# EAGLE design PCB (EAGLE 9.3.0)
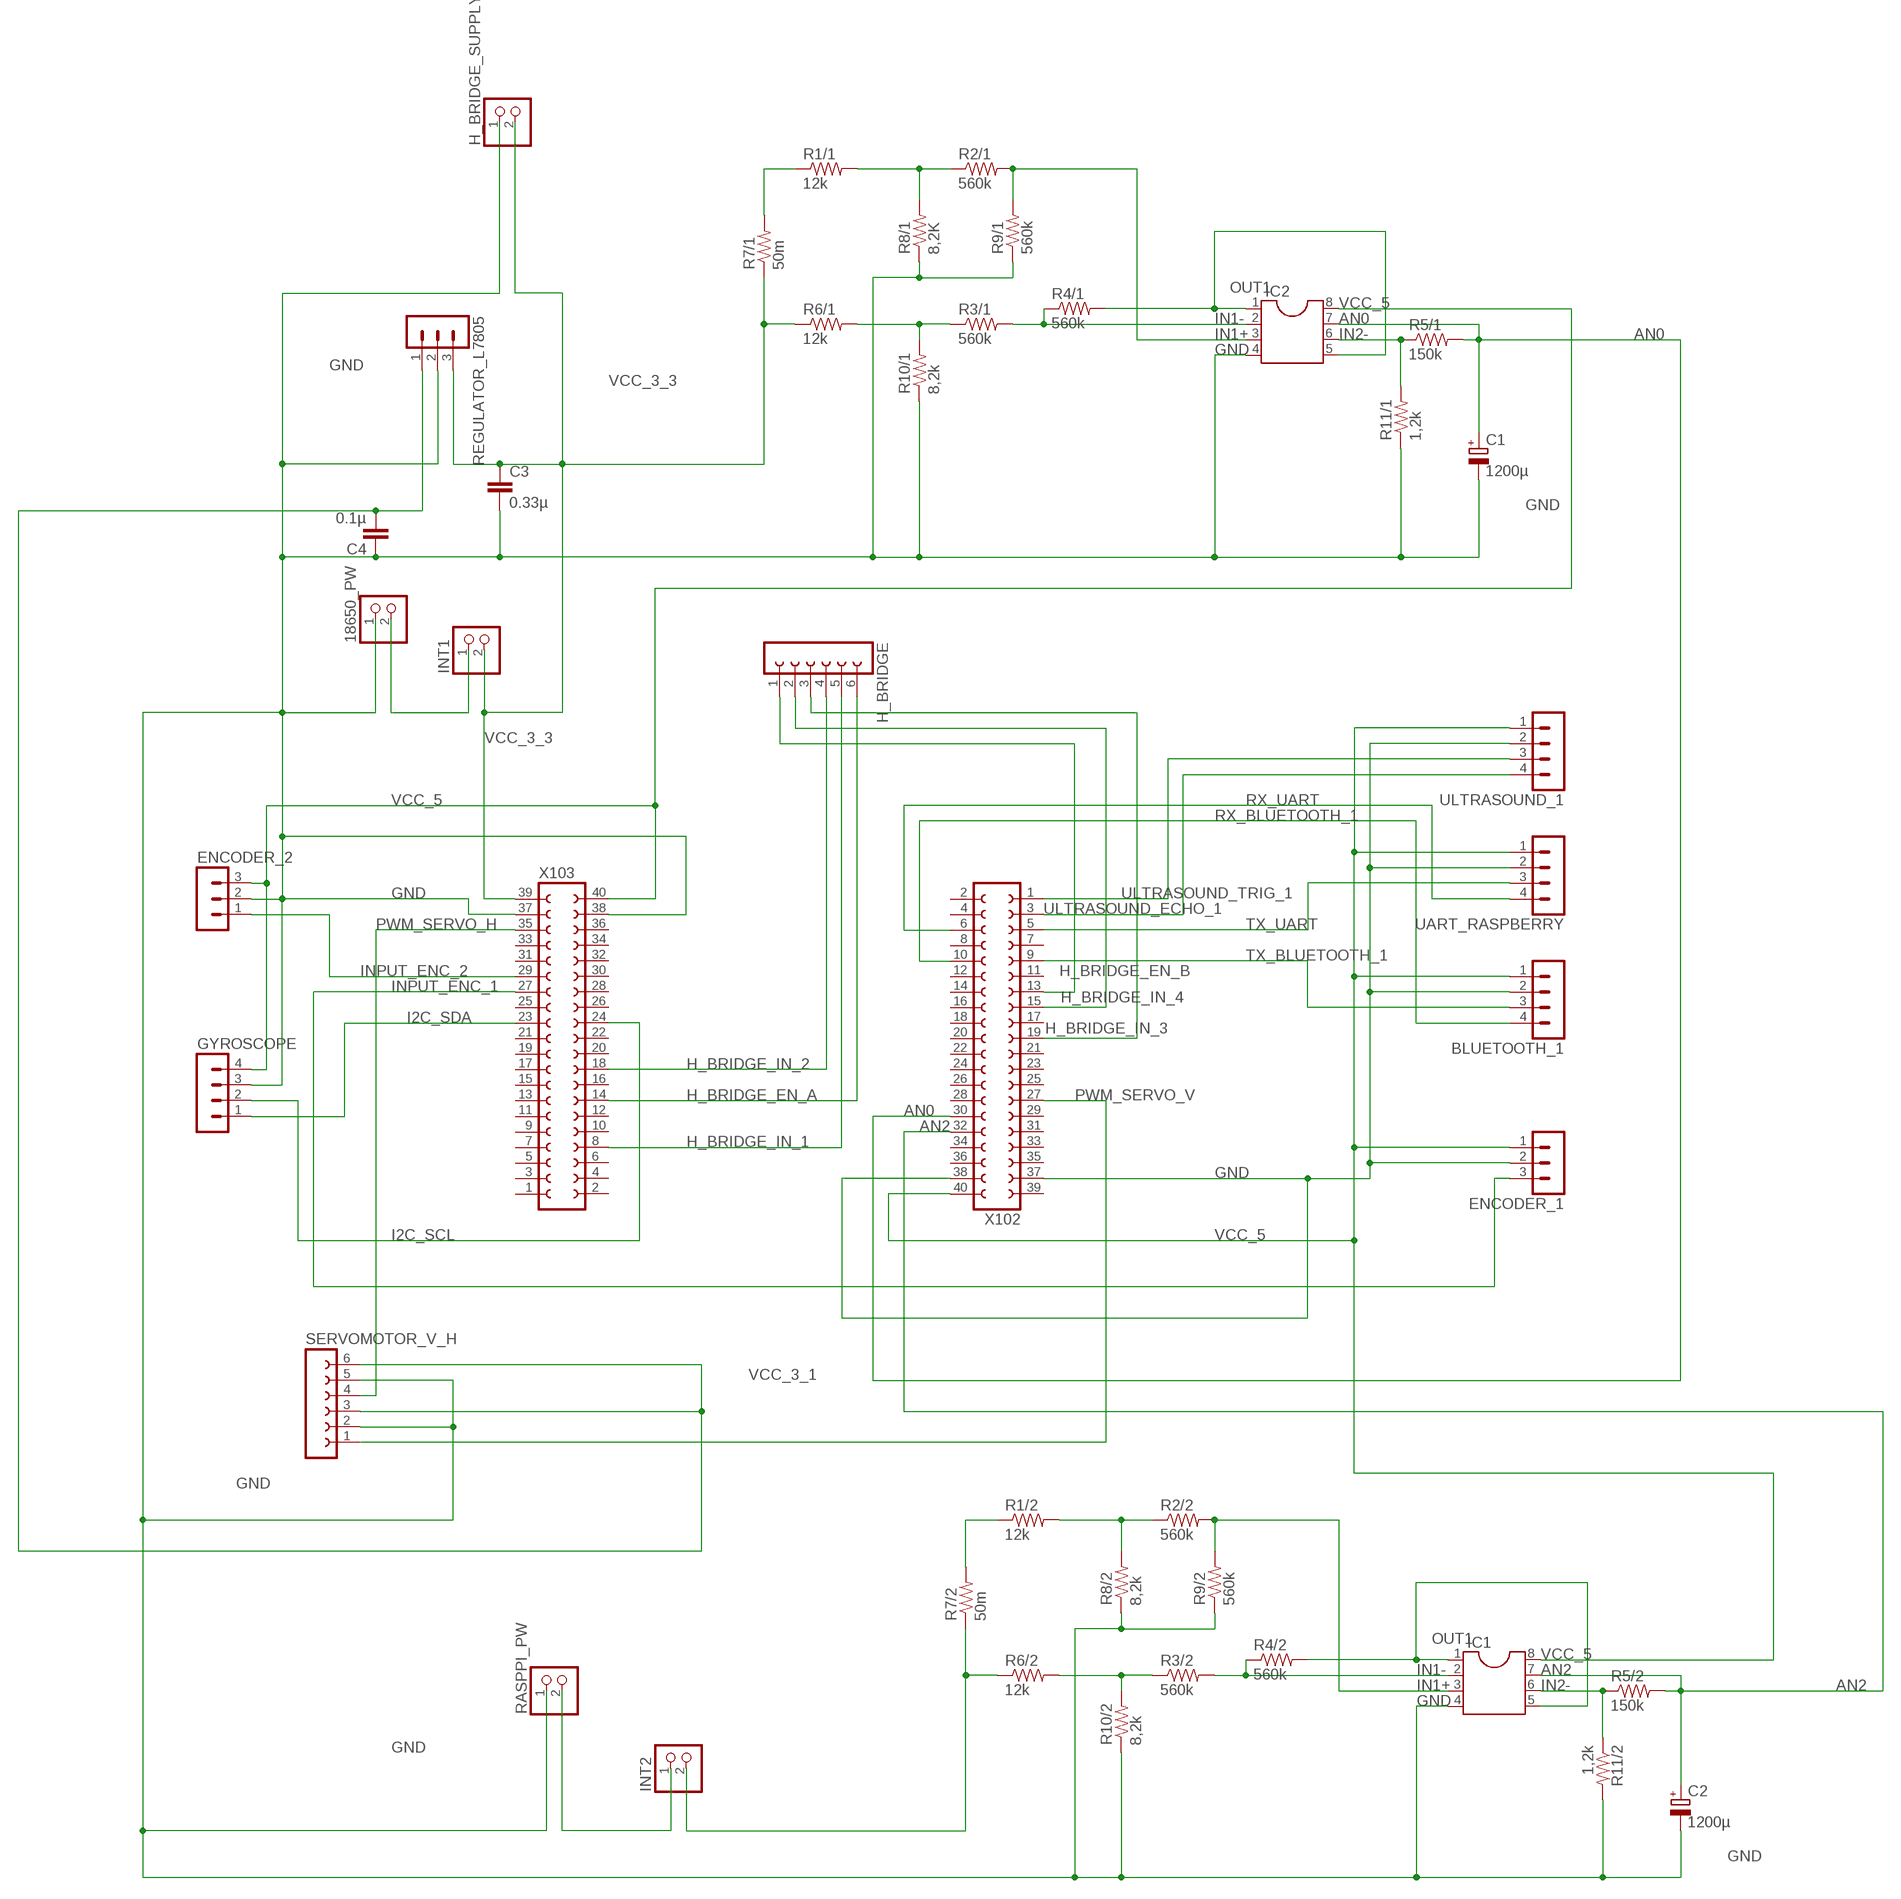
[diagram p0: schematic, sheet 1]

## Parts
18650_PW  PINHD-1X2  [1X02]
BLUETOOTH_1  MA04-1  [MA04-1]
C1  1200µ  CPOL-EUE2-5  [E2-5]
C2  1200µ  CPOL-EUE2-5  [E2-5]
C3  0.33µ  C-EU025-025X050  [C025-025X050]
C4  0.1µ  C-EU025-025X050  [C025-025X050]
ENCODER_1  MA03-1  [MA03-1]
ENCODER_2  MA03-1  [MA03-1]
GYROSCOPE  MA04-1  [MA04-1]
H_BRIDGE  FE06-1  [FE06]
H_BRIDGE_SUPPLY  PINHD-1X2  [1X02]
IC1  DIL8  [DIL08]
IC2  DIL8  [DIL08]
INT1  PINHD-1X2  [1X02]
INT2  PINHD-1X2  [1X02]
R1/1  12k  R-US_0207/10  [0207/10]
R1/2  12k  R-US_0207/10  [0207/10]
R2/1  560k  R-US_0207/10  [0207/10]
R2/2  560k  R-US_0207/10  [0207/10]
R3/1  560k  R-US_0207/10  [0207/10]
R3/2  560k  R-US_0207/10  [0207/10]
R4/1  560k  R-US_0207/10  [0207/10]
R4/2  560k  R-US_0207/10  [0207/10]
R5/1  150k  R-US_0207/10  [0207/10]
R5/2  150k  R-US_0207/10  [0207/10]
R6/1  12k  R-US_0207/10  [0207/10]
R6/2  12k  R-US_0207/10  [0207/10]
R7/1  50m  R-US_0207/10  [0207/10]
R7/2  50m  R-US_0207/10  [0207/10]
R8/1  8,2K  R-US_0207/10  [0207/10]
R8/2  8,2k  R-US_0207/10  [0207/10]
R9/1  560k  R-US_0207/10  [0207/10]
R9/2  560k  R-US_0207/10  [0207/10]
R10/1  8,2k  R-US_0207/10  [0207/10]
R10/2  8,2k  R-US_0207/10  [0207/10]
R11/1  1,2k  R-US_0207/10  [0207/10]
R11/2  1,2k  R-US_0207/10  [0207/10]
RASPPI_PW  PINHD-1X2  [1X02]
REGULATOR_L7805  MA03-1  [MA03-1]
SERVOMOTOR_V_H  FE06-1  [FE06]
UART_RASPBERRY  MA04-1  [MA04-1]
ULTRASOUND_1  MA04-1  [MA04-1]
X102  FE20-2  [FE20-2]
X103  FE20-2  [FE20-2]

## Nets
AN0: C1.+ IC2.7 R5/1.2 X102.30
AN2: C2.+ IC1.7 R5/2.2 X102.32
GND: 18650_PW.1 BLUETOOTH_1.2 C1.- C2.- C3.2 C4.1 ENCODER_1.2 ENCODER_2.2 GYROSCOPE.3 H_BRIDGE_SUPPLY.1 IC1.4 IC2.4 R8/1.1 R8/2.1 R9/1.1 R9/2.1 R10/1.1 R10/2.1 R11/1.1 R11/2.2 RASPPI_PW.1 REGULATOR_L7805.2 SERVOMOTOR_V_H.2 SERVOMOTOR_V_H.5 UART_RASPBERRY.2 ULTRASOUND_1.2 X102.37 X102.38 X103.37 X103.38
H_BRIDGE_EN_A: H_BRIDGE.6 X103.14
H_BRIDGE_EN_B: H_BRIDGE.1 X102.13
H_BRIDGE_IN_1: H_BRIDGE.5 X103.8
H_BRIDGE_IN_2: H_BRIDGE.4 X103.18
H_BRIDGE_IN_3: H_BRIDGE.3 X102.19
H_BRIDGE_IN_4: H_BRIDGE.2 X102.15
I2C_SCL: GYROSCOPE.2 X103.24
I2C_SDA: GYROSCOPE.1 X103.23
IN1+: IC1.3 IC2.3 R2/1.2 R2/2.2 R9/1.2 R9/2.2
IN1-: IC1.2 IC2.2 R3/1.2 R3/2.2 R4/1.1 R4/2.1
IN2-: IC1.6 IC2.6 R5/1.1 R5/2.1 R11/1.2 R11/2.1
INPUT_ENC_1: ENCODER_1.3 X103.27
INPUT_ENC_2: ENCODER_2.1 X103.29
N$1: R3/1.1 R6/1.2 R10/1.2
N$2: R3/2.1 R6/2.2 R10/2.2
N$3: R1/1.1 R7/1.2
N$4: R1/1.2 R2/1.1 R8/1.2
N$5: R1/2.1 R7/2.2
N$6: R1/2.2 R2/2.1 R8/2.2
N$7: INT2.2 R6/2.1 R7/2.1
N$8: INT2.1 RASPPI_PW.2
N$9: 18650_PW.2 INT1.1
OUT1: IC1.1 IC1.5 IC2.1 IC2.5 R4/1.2 R4/2.2
PWM_SERVO_H: SERVOMOTOR_V_H.4 X103.35
PWM_SERVO_V: SERVOMOTOR_V_H.1 X102.27
RX_BLUETOOTH_1: BLUETOOTH_1.4 X102.10
RX_UART: UART_RASPBERRY.4 X102.6
TX_BLUETOOTH_1: BLUETOOTH_1.3 X102.9
TX_UART: UART_RASPBERRY.3 X102.5
ULTRASOUND_ECHO_1: ULTRASOUND_1.4 X102.3
ULTRASOUND_TRIG_1: ULTRASOUND_1.3 X102.1
VCC_3_1: C4.2 REGULATOR_L7805.1 SERVOMOTOR_V_H.3 SERVOMOTOR_V_H.6
VCC_3_3: C3.1 H_BRIDGE_SUPPLY.2 INT1.2 R6/1.1 R7/1.1 REGULATOR_L7805.3 X103.39
VCC_5: BLUETOOTH_1.1 ENCODER_1.1 ENCODER_2.3 GYROSCOPE.4 IC1.8 IC2.8 UART_RASPBERRY.1 ULTRASOUND_1.1 X102.40 X103.40
Unconnected: X102.2 X102.4 X102.7 X102.8 X102.11 X102.12 X102.14 X102.16 X102.17 X102.18 X102.20 X102.21 X102.22 X102.23 X102.24 X102.25 X102.26 X102.28 X102.29 X102.31 X102.33 X102.34 X102.35 X102.36 X102.39 X103.1 X103.2 X103.3 X103.4 X103.5 X103.6 X103.7 X103.9 X103.10 X103.11 X103.12 X103.13 X103.15 X103.16 X103.17 X103.19 X103.20 X103.21 X103.22 X103.25 X103.26 X103.28 X103.30 X103.31 X103.32 X103.33 X103.34 X103.36

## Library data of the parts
18650_PW H_BRIDGE_SUPPLY INT1 INT2 RASPPI_PW = pinhead:PINHD-1X2: PIN HEADER
BLUETOOTH_1 GYROSCOPE UART_RASPBERRY ULTRASOUND_1 = con-lstb:MA04-1: PIN HEADER; OC_FARNELL: unknown; OC_NEWARK: unknown
C1 C2 = rcl:CPOL-EU: POLARIZED CAPACITOR, European symbol; SPICEPREFIX: C
C3 C4 = rcl:C-EU: CAPACITOR, European symbol; SPICEPREFIX: C
ENCODER_1 ENCODER_2 REGULATOR_L7805 = con-lstb:MA03-1: PIN HEADER; OC_FARNELL: unknown; OC_NEWARK: unknown
H_BRIDGE SERVOMOTOR_V_H = con-lsta:FE06-1: FEMALE HEADER; OC_FARNELL: unknown; OC_NEWARK: unknown
IC1 IC2 = ic-package:DIL8: Dual In Line / Socket
R1/1 R1/2 R2/1 R2/2 R3/1 R3/2 R4/1 R4/2 R5/1 R5/2 R6/1 R6/2 R7/1 R7/2 R8/1 R8/2 R9/1 R9/2 R10/1 R10/2 R11/1 R11/2 = rcl:R-US_: RESISTOR, American symbol; SPICEPREFIX: R
X102 X103 = con-lsta:FE20-2: FEMALE HEADER; OC_FARNELL: unknown; OC_NEWARK: unknown

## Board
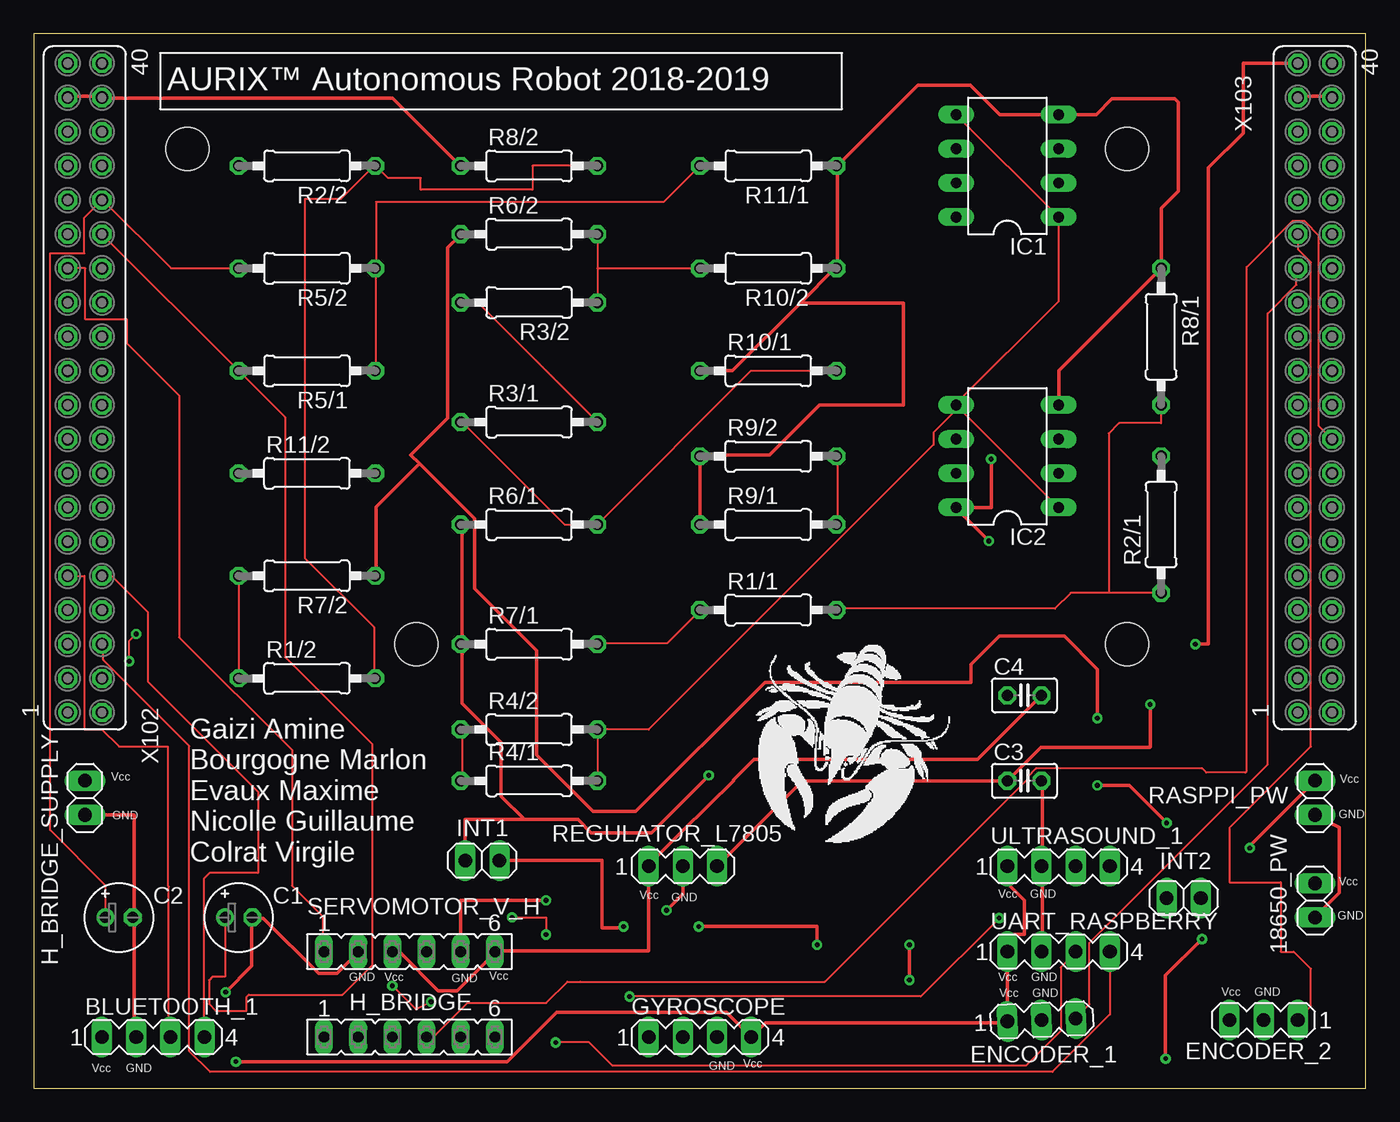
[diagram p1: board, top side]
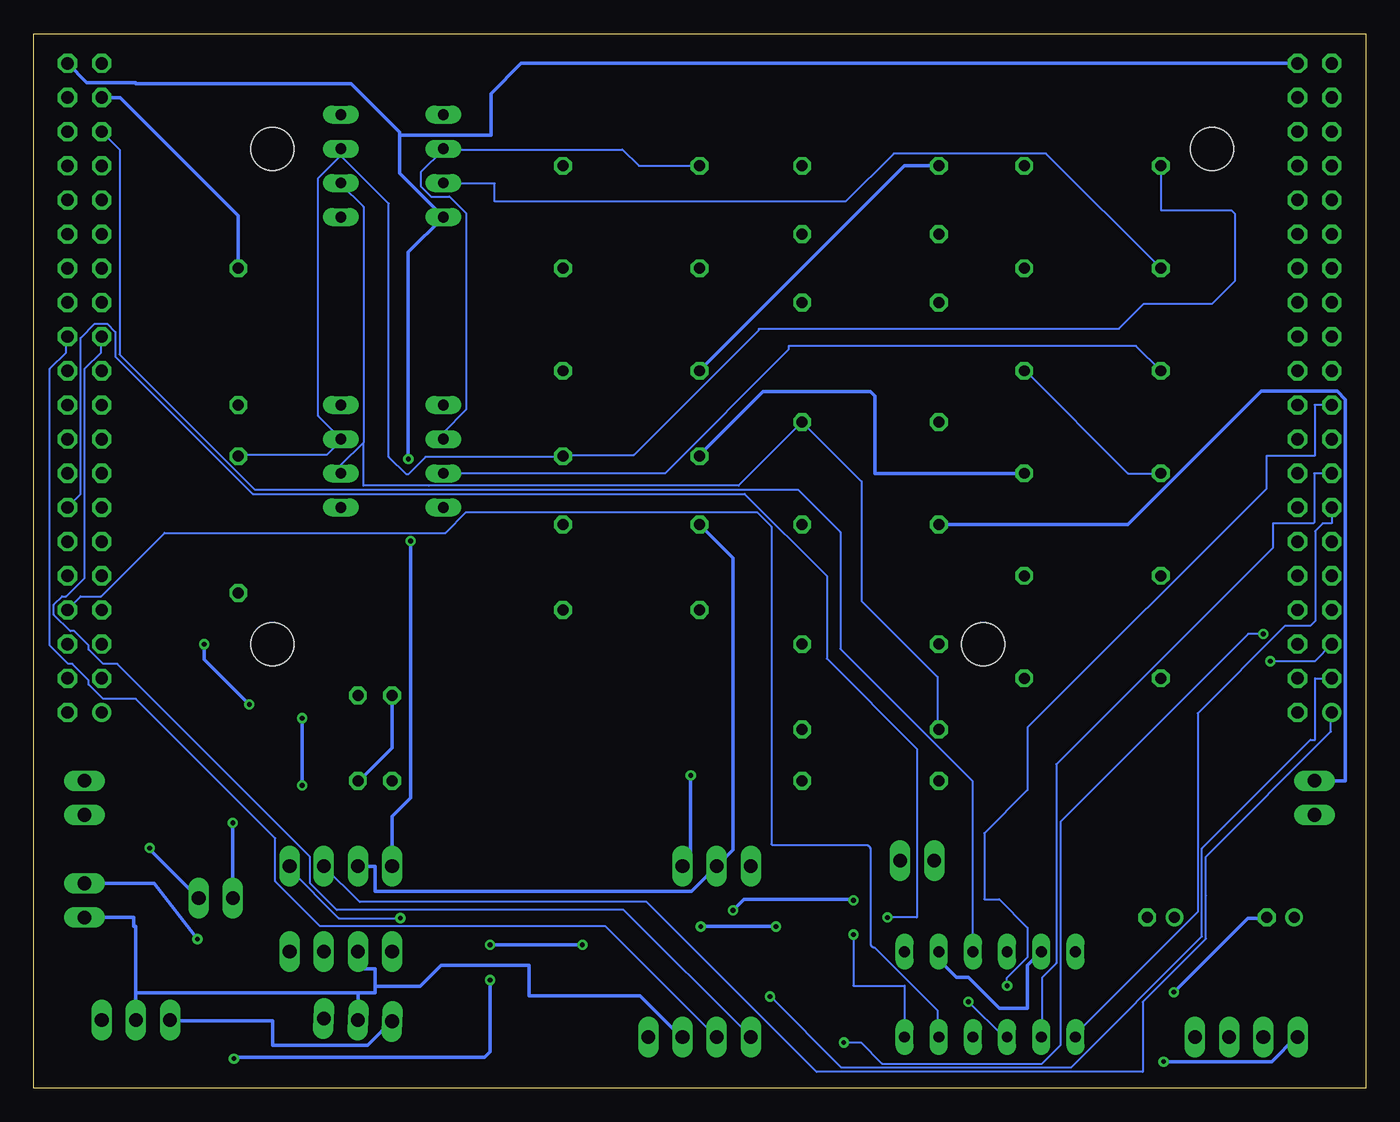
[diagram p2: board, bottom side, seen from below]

Size 99.04 x 78.41 mm. Coordinates in mm from the lower left corner, seen from the top.
Outline: 0,0 99.04,0 99.04,78.41 0,78.41 0,0
Copper layers (1*16): Top 0.035mm / dielectric 1.5mm / Bottom 0.035mm
Design rules "default": minimum track width 6mil, minimum drill 0.35mm, track to track 6mil, track to pad 6mil, pad to pad 6mil, via to via 6mil, smd to smd 6mil, copper to edge 40mil, drill to drill 6mil, minimum pad ring 10mil, minimum via ring 8mil, stop-mask expansion 4mil, vias tented up to drill 0mil, thermal gap 10mil
Holes 3.2 mm at 11.43,69.85 81.28,69.85 28.45,33.02 81.28,33.02

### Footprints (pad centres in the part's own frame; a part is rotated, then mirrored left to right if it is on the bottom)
1X02 = drill 1.016 long: 1 -1.27,0; 2 1.27,0
MA04-1 = drill 1.016 long: 1 -3.81,0; 2 -1.27,0; 3 1.27,0; 4 3.81,0
E2-5 = drill 0.813 pad 1.27: + -1.016,0 | drill 0.813 pad 1.27 octagon: - 1.016,0
C025-025X050 = drill 0.813 octagon: 1 -1.27,0; 2 1.27,0
MA03-1 = drill 1.016 long: 1 -2.54,0; 2 0,0; 3 2.54,0
FE06 = drill 0.813 long: 1 -6.35,0; 2 -3.81,0; 3 -1.27,0; 4 1.27,0; 5 3.81,0; 6 6.35,0
DIL08 = drill 0.813 long: 1 -3.81,-3.81; 2 -1.27,-3.81; 3 1.27,-3.81; 4 3.81,-3.81; 5 3.81,3.81; 6 1.27,3.81; 7 -1.27,3.81; 8 -3.81,3.81
0207/10 = drill 0.813 octagon: 1 -5.08,0; 2 5.08,0
FE20-2 = drill 0.914: 1 -24.13,1.27 | drill 0.914 octagon: 2 -24.13,-1.27; 3 -21.59,1.27; 4 -21.59,-1.27; 5 -19.05,1.27; 6 -19.05,-1.27; 7 -16.51,1.27; 8 -16.51,-1.27; 9 -13.97,1.27; 10 -13.97,-1.27; 11 -11.43,1.27; 12 -11.43,-1.27; 13 -8.89,1.27; 14 -8.89,-1.27; 15 -6.35,1.27; 16 -6.35,-1.27; 17 -3.81,1.27; 18 -3.81,-1.27; 19 -1.27,1.27; 20 -1.27,-1.27; 21 1.27,1.27; 22 1.27,-1.27; 23 3.81,1.27; 24 3.81,-1.27; 25 6.35,1.27; 26 6.35,-1.27; 27 8.89,1.27; 28 8.89,-1.27; 29 11.43,1.27; 30 11.43,-1.27; 31 13.97,1.27; 32 13.97,-1.27; 33 16.51,1.27; 34 16.51,-1.27; 35 19.05,1.27; 36 19.05,-1.27; 37 21.59,1.27; 38 21.59,-1.27; 39 24.13,1.27; 40 24.13,-1.27

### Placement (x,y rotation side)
18650_PW  95.25,13.97 90 top
BLUETOOTH_1  8.89,3.81 0 top
C1  15.24,12.7 0 top
C2  6.35,12.7 0 top
C3  73.66,22.86 0 top
C4  73.66,29.21 0 top
ENCODER_1  74.93,5.08 2.4 top
ENCODER_2  91.44,5.08 180 top
GYROSCOPE  49.53,3.81 0 top
H_BRIDGE  27.94,3.81 0 top
H_BRIDGE_SUPPLY  3.81,21.59 90 top
IC1  72.39,68.58 90 top
IC2  72.39,46.99 90 top
INT1  33.36,16.93 180 top
INT2  85.5,14.14 180 top
R1/1  54.61,35.56 0 top
R1/2  20.32,30.48 0 top
R2/1  83.82,41.91 90 top
R2/2  20.32,68.58 180 top
R3/1  36.83,49.53 0 top
R3/2  36.83,58.42 180 top
R4/1  36.83,22.86 0 top
R4/2  36.83,26.67 0 top
R5/1  20.32,53.34 180 top
R5/2  20.32,60.96 180 top
R6/1  36.83,41.91 0 top
R6/2  36.83,63.5 0 top
R7/1  36.83,33.02 0 top
R7/2  20.32,38.1 180 top
R8/1  83.82,55.88 270 top
R8/2  36.83,68.58 0 top
R9/1  54.61,41.91 0 top
R9/2  54.61,46.99 0 top
R10/1  54.61,53.34 0 top
R10/2  54.61,60.96 180 top
R11/1  54.61,68.58 180 top
R11/2  20.32,45.72 0 top
RASPPI_PW  95.25,21.59 90 top
REGULATOR_L7805  48.26,16.51 0 top
SERVOMOTOR_V_H  27.94,10.16 0 top
UART_RASPBERRY  76.2,10.16 0 top
ULTRASOUND_1  76.2,16.51 0 top
X102  3.81,52.07 90 top
X103  95.25,52.07 90 top

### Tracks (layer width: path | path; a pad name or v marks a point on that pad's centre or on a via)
AN0
  Top 0.152: X102.30 R5/1.2 18.69,49.89 18.69,32.05 25.15,25.6 25.15,9.14 22.96,6.96 16,6.96 15.83,6.79 15.83,5.76 13.54,5.76 13.04,6.26 13.04,8.04 13.29,8.3 14.22,8.3 C1.+
  Bottom 0.152: IC2.7 52.12,45.72 42.92,54.92 42.92,55.2 17.1,55.2 R5/1.2
AN2
  Top 0.152: C2.+ 5.33,15.09 1.22,19.2 1.22,62.07 3.77,62.07 3.77,64.73 X102.32 5.18,65.99 10.21,60.96 R5/2.2
  Bottom 0.152: IC1.7 68.53,67.26 64.76,67.26 64.76,65.92 38.68,65.92 35.1,69.49 23.77,69.49 R5/2.2
GND  (via drill 0.35)
  Top 0.254: X103.37 94.03,73.76 96.47,73.76 X103.38 | IC2.4 76.2,53.34 R8/1.1 83.82,65.43 85.08,66.69 85.08,73.31 84.83,73.57 80.17,73.57 78.99,72.39 IC1.4 71.83,72.39 69.65,74.57 65.73,74.57 59.74,68.58 | X102.37 2.59,73.76 5.03,73.76 X102.38 5.18,73.61 26.67,73.61 31.7,68.58 R8/2.1 | R10/1.1 51.97,53.34 57.01,58.38 | 57.01,58.38 59.59,60.96 R10/2.1 59.74,60.96 59.74,68.58 | 59.74,68.58 R11/1.1 | C3.2 74.98,22.86 74.98,16.61 ULTRASOUND_1.2 74.98,16.46 74.98,10.21 UART_RASPBERRY.2 | 7.47,12.65 7.47,3.96 BLUETOOTH_1.2 | 7.47,12.65 C2.- | SERVOMOTOR_V_H.2 24.08,10.06 22.55,8.53 21.18,8.53 17.07,12.65 16.31,12.65 C1.- 16.22,12.73 16.22,9.09 v14.28,7.15 | R9/1.1 R9/2.1 49.53,47.09 54.71,47.09 58.42,50.8 64.68,50.8 64.68,58.38 57.01,58.38 | REGULATOR_L7805.2 48.26,14.44 v47.05,13.23 | 18650_PW.1 97.08,14.53 97.08,19.41 RASPPI_PW.1 | SERVOMOTOR_V_H.5 31.75,13.97 v38.1,13.97 | 7.47,12.65 7.47,20.32 H_BRIDGE_SUPPLY.1
  Bottom 0.254: X103.37 92.61,73.66 83.82,64.87 R8/1.1 | R8/2.1 34.29,68.58 R10/1.1 | 91.44,6.71 ENCODER_2.2 91.44,7.11 | C4.1 72.39,25.3 74.83,22.86 C3.2 | GYROSCOPE.3 50.9,3.81 53.95,6.86 62.22,6.86 62.22,9.14 68.74,9.14 70.31,7.58 73.66,7.58 | UART_RASPBERRY.2 74.83,10.06 74.83,8.89 73.66,8.89 73.66,7.58 | 74.93,7.11 73.66,7.11 73.66,7.58 | 74.93,7.11 91.44,7.11 | SERVOMOTOR_V_H.2 25.15,9.14 25.15,5.94 27.26,5.94 29.56,8.24 30.44,8.24 31.7,9.5 31.7,10.06 SERVOMOTOR_V_H.5 | v14.28,7.15 8.77,12.65 7.47,12.65 C2.- | R11/2.2 36.49,45.72 36.49,51.47 36.83,51.81 44.81,51.81 49.53,47.09 R9/2.1 | R9/1.1 47.04,39.42 47.04,17.73 REGULATOR_L7805.2 50.14,14.63 73.66,14.63 73.66,16.51 ULTRASOUND_1.2 | v47.05,13.23 46.23,14.05 38.19,14.05 v38.1,13.97 | 18650_PW.1 91.6,12.7 91.6,12.02 91.44,12.02 91.44,7.11 | ENCODER_1.2 74.93,7.11
H_BRIDGE_EN_A  (via drill 0.35)
  Top 0.152: v35.56,12.7 38.1,12.7 v38.1,11.43
  Bottom 0.152: 92.96,56.24 92.96,54.41 82.75,44.2 46.18,44.2 40.08,38.1 40.08,31.95 33.38,25.25 33.38,12.7 v35.56,12.7 | 92.96,56.24 93.57,56.84 94.49,56.84 95.56,55.78 95.56,44.2 96.47,43.28 X103.14 | v38.1,11.43 38.1,7.62 34.29,7.62 H_BRIDGE.6 | 92.96,56.24
H_BRIDGE_EN_B
  Bottom 0.152: H_BRIDGE.1 21.49,3.81 21.49,4.12 12.5,13.11 12.5,27.89 6.01,34.37 4.15,34.37 3.78,34.74 3.78,41.43 3.22,41.99 2.54,41.99 X102.13
H_BRIDGE_IN_1
  Bottom 0.152: H_BRIDGE.5 31.85,3.81 31.85,5.79 36.52,10.46 arc90 36.83,10.77 36.83,17.78 arc-90 37.13,18.09 44.15,18.09 44.2,18.14 44.2,41.76 45.26,42.82 66.9,42.82 68.43,41.3 89.31,41.3 94.03,36.58 95.56,36.58 96.47,35.66 X103.8
H_BRIDGE_IN_2
  Top 0.152: H_BRIDGE.4 29.72,3.81 32.26,6.35 38.1,6.35 39.67,7.92 40.64,7.92 58.83,7.92 73.91,23.01 73.91,23.16 74.52,23.77 86.87,23.77 87.17,23.47 90.07,23.47 90.17,23.57 90.17,61.06 | 90.17,61.06 93.57,64.47 94.49,64.47 95.56,63.4 95.56,62.82 | 95.56,62.82 95.56,49.23 X103.18 | 95.56,62.82 | 90.17,61.06
H_BRIDGE_IN_3  (via drill 0.35)
  Top 0.152: v29.55,6.43 28.42,5.87 v26.67,7.62
  Bottom 0.152: v29.55,6.43 26.92,3.81 H_BRIDGE.3 | v26.67,7.62 26.67,8.23 25.15,9.75 25.15,11.94 27.26,14.05 28.36,14.05 28.36,18.97 25.15,22.18 25.15,26.82 7.4,44.57 7.4,47.01 3.8,47.01 3.8,50.8 X102.19
H_BRIDGE_IN_4
  Bottom 0.152: H_BRIDGE.2 24.08,3.81 24.08,8.23 23.01,9.3 23.01,24.08 6.91,40.18 6.91,41.99 3.89,41.99 3.84,42.05 3.84,45.72 X102.15
I2C_SCL
  Bottom 0.152: X103.24 96.62,55.78 96.62,54.71 97.84,53.49 97.84,32.92 96.47,31.55 96.16,31.55 94.94,30.33 94.94,30.02 93.88,28.96 91.44,28.96 81.08,18.59 81.08,15.39 77.72,12.04 56.54,12.04 48.31,3.81 GYROSCOPE.2
I2C_SDA
  Bottom 0.152: 97.54,35.2 97.54,35.97 96.93,36.58 96.62,36.58 95.25,37.95 95.25,53.49 94.03,54.71 94.03,55.78 X103.23 | 97.54,35.2 96.32,33.98 96.01,33.98 94.94,32.92 94.94,32.61 93.88,31.55 92.81,31.55 78.49,17.22 78.49,15.24 76.5,13.26 55.17,13.26 GYROSCOPE.1 | 97.54,35.2
IN1+
  Top 0.152: R9/1.2 59.74,41.91 59.74,46.94 R9/2.2
  Bottom 0.152: R2/1.2 83.82,47.09 77.27,47.09 76.2,48.16 IC2.3 76.2,48.31 77.88,49.99 77.88,67.67 76.2,69.34 | 76.2,69.34 IC1.3 76.2,69.8 | R2/2.2 15.24,65.27 9.99,65.27 9.74,65.02 9.74,60.02 11.43,58.33 16.5,58.33 18.36,56.47 45.12,56.47 45.12,56.38 54.41,47.09 59.59,47.09 R9/2.2 59.74,46.94 69.93,46.94 69.93,46.9 71.2,45.63 71.33,45.63 72.64,46.94 72.64,65.78 76.2,69.34
IN1-
  Top 0.152: R4/1.1 31.85,22.91 31.85,26.67 R4/2.1 | R3/1.2 33.07,58.37 31.85,58.37 R3/2.2
  Bottom 0.152: IC2.2 76.2,46.33 74.52,48.01 | 74.52,48.01 74.52,65.53 76.2,67.21 IC1.2 | R4/2.1 31.85,26.67 31.85,30.58 37.49,36.22 37.49,45.11 R3/1.2 46.63,44.81 69.65,44.81 74.52,44.81 74.52,48.01
IN2-
  Top 0.152: 25.45,60.96 25.45,53.34 R5/1.1 | R11/1.2 46.84,65.89 25.45,65.89 25.45,60.96 | R5/2.1 25.45,60.96
  Bottom 0.152: R11/2.1 17.68,45.72 25.3,53.34 R5/1.1 | IC2.6 68.58,48.77 66.9,50.44 66.9,65.08 68.12,66.29 69.49,66.29 70.26,67.06 70.26,68.12 68.58,69.8 | R11/1.2 54.05,68.58 55.27,69.8 68.58,69.8 | 68.58,69.8 IC1.6
INPUT_ENC_1
  Top 0.152: X103.27 93.88,60.96 93.88,59.74 91.75,57.61 91.75,24.08 78.49,10.82 78.49,6.25 77.57,5.33 ENCODER_1.3
INPUT_ENC_2
  Top 0.152: X103.29 94.03,63.4 94.03,62.33 94.94,61.42 94.94,25.4 88.9,19.36 88.9,15.32 92.7,15.32 92.7,10.16 93.67,10.16 94.94,8.89 94.94,6.1 94.03,5.18 ENCODER_2.1
N$1
  Top 0.152: R3/1.1 31.85,49.53 39.47,41.91 R6/1.2 53.34,53.34 R10/1.2
N$2
  Top 0.152: R6/2.2 41.91,60.96 | 41.91,60.96 R3/2.1 | 41.91,60.96 R10/2.2
N$3
  Top 0.152: R7/1.2 41.91,33.07 47.09,33.07 49.53,35.51 R1/1.1
N$4
  Top 0.152: R1/1.2 59.74,35.66 75.94,35.66 77.11,36.83 79.92,36.83 | R8/1.2 83.82,49.44 80.68,49.44 79.92,48.68 79.92,36.83 | 83.82,36.88 R2/1.1 79.92,36.83
N$5
  Top 0.152: R7/2.2 R1/2.1
N$6
  Top 0.152: R1/2.2 25.3,30.48 25.3,34.29 20.15,39.44 20.15,66.12 22.84,66.12 25.3,68.58 R2/2.1 25.45,68.58 26.36,67.67 28.78,67.67 28.78,66.8 37.08,66.8 37.08,68.58 R8/2.2
N$7  (via drill 0.35)
  Top 0.254: 28.68,46.46 25.45,43.23 25.45,38.1 R7/2.1 | R6/2.1 31.7,63.4 30.79,62.48 30.79,49.84 28.04,47.09 28.68,46.46 | 28.68,46.46 32.77,42.37 32.77,37.16 37.4,32.53 37.4,24.78 41.6,20.57 44.76,20.57 54.36,30.18 69.67,30.18 69.67,31.49 71.79,33.61 76.62,33.61 79.07,31.15 79.07,30.18 v79.07,27.51 | v84.23,19.73 81.44,22.52 v79.07,22.52
  Bottom 0.152: v84.23,19.73
  Bottom 0.254: INT2.2 v84.23,19.73 | v79.07,22.52 v79.07,27.51
N$8  (via drill 0.35)
  Top 0.152: v90.42,17.86 90.42,18.02
  Top 0.254: 90.42,18.02 RASPPI_PW.2
  Bottom 0.152: 90.42,17.78 v90.42,17.86
  Bottom 0.254: INT2.1 90.42,17.78
N$9  (via drill 0.35)
  Top 0.152: 43.85,11.94 v43.85,12.02
  Top 0.254: INT1.1 42.24,16.93 42.24,11.94 43.85,11.94 | v49.44,12.02 58.24,12.02 v58.24,10.67 | v65.1,10.67 v65.1,8.04 | v84.15,2.2 84.15,8.38 v86.86,11.09
  Bottom 0.152: 84.07,2.29 v84.15,2.2 | 18650_PW.2
  Bottom 0.254: v43.85,12.02 v49.44,12.02 | v65.1,10.67 v58.24,10.67 | v65.1,8.04 65.1,2.71 65.53,2.29 84.07,2.29 | v86.86,11.09 90.08,15.24 18650_PW.2
OUT1
  Top 0.152: IC1.5 IC1.1 76.2,58.52 68.58,50.9 IC2.5 | R4/1.2 R4/2.2 45.72,26.67 66.9,47.85 66.9,48.77 68.73,50.6 | 68.73,50.6 76.2,43.13 IC2.1 | 68.73,50.6 68.58,50.75 IC2.5 | 68.73,50.6 IC2.5
PWM_SERVO_H
  Bottom 0.152: X103.35 92.66,69.8 92.66,54.56 82.6,44.5 42.22,44.5 39.06,41.35 39.06,32.66 29.26,22.86 29.26,10.21 SERVOMOTOR_V_H.4
PWM_SERVO_V
  Top 0.152: SERVOMOTOR_V_H.1 21.49,10.21 21.49,12.78 19.21,15.06 19.21,25.14 10.82,33.53 10.82,51.51 6.95,55.38 6.95,57.16 3.84,57.16 3.84,60.96 X102.27
RX_BLUETOOTH_1
  Top 0.152: X102.10 5.79,38.1 8.48,35.41 8.48,30.24 16.68,22.05 16.68,16 13.07,16 12.65,15.58 12.65,3.81 BLUETOOTH_1.4
RX_UART
  Top 0.152: UART_RASPBERRY.4 80.01,5.49 75.74,1.22 13.11,1.22 11.58,2.74 11.58,25.45 5.18,31.85 5.18,32.92 X102.6
TX_BLUETOOTH_1
  Top 0.152: BLUETOOTH_1.3 10.06,3.81 10.06,14.99 9.98,15.06 9.98,25.4 6.35,25.4 5.08,26.67 3.78,26.67 3.78,38.1 X102.9
TX_UART  (via drill 0.35)
  Top 0.152: v38.81,3.4 41.3,3.4 43.03,1.68 73.76,1.68 76.35,4.27 76.35,8.99 77.42,10.06 UART_RASPBERRY.3 | v7.11,31.75 7.11,33.27 v7.62,33.78
  Bottom 0.152: v38.81,3.4 37.54,3.4 35.97,1.83 24.08,1.83 22.71,3.2 22.71,19.81 8.74,33.78 v7.62,33.78 | X102.5 3.81,31.75 v7.11,31.75
ULTRASOUND_ECHO_1  (via drill 0.35)
  Top 0.152: v44.3,6.82 65.95,6.82 v71.78,12.65
  Bottom 0.152: v44.3,6.82 44.28,6.82 38.98,1.52 21.95,1.52 12.19,11.28 12.19,17.83 4.12,25.91 3.78,25.91 3.78,30.48 X102.3 | v71.78,12.65 76.35,12.65 80.01,16.31 ULTRASOUND_1.4
ULTRASOUND_TRIG_1
  Bottom 0.152: X102.1 2.59,27.89 2.59,26.52 11.89,17.22 11.89,14.31 11.89,11.12 16.59,6.43 16.59,1.22 40.84,1.22 53.47,13.84 74.8,13.84 ULTRASOUND_1.3
VCC_3_1
  Top 0.254: SERVOMOTOR_V_H.3 26.67,10.06 27.28,10.06 30.07,7.26 31.5,7.26 34.29,10.06 SERVOMOTOR_V_H.6 34.29,10.21 45.72,10.21 REGULATOR_L7805.1 45.72,16.61 48.21,19.1 52.02,22.86 52.02,22.91 53.54,24.43 70.16,24.43 C4.2
VCC_3_3  (via drill 0.35)
  Top 0.254: R6/1.1 31.85,41.91 31.85,33.07 R7/1.1 31.85,32.92 31.85,28.6 34.76,25.7 34.76,21.71 36.49,19.98 | REGULATOR_L7805.3 57.15,22.86 C3.1 74.88,25.35 82.97,25.35 83.01,25.39 83.01,25.74 v83.01,28.53 | v50.19,23.27 45.92,19 41.45,19 40.47,19.98 36.49,19.98 | v86.36,33.02 87.33,33.02 87.33,68.43 89.92,71.02 89.92,76.2 X103.39 | INT1.2 32.09,19.73 | 32.09,19.73 32.09,19.98 | 32.09,19.98 36.49,19.98 | 32.09,19.98 32.09,19.73 | 32.09,19.73
  Bottom 0.254: R6/1.1 17.68,41.91 7.77,51.82 2.13,51.82 1.52,51.21 1.52,22.86 H_BRIDGE_SUPPLY.2 | v50.19,23.27 50.19,17.17 50.75,16.61 REGULATOR_L7805.3 | v86.36,33.02 86.36,31.89 v83.01,28.53
VCC_5  (via drill 0.35)
  Top 0.254: ULTRASOUND_1.1 72.39,15.24 73.66,13.97 73.66,11.43 72.39,11.43 UART_RASPBERRY.1 72.39,5.03 ENCODER_1.1 72.39,4.88 54.41,4.88 GYROSCOPE.4 51.51,5.64 38.86,5.64 35.2,1.98 v15.04,1.98 | v71.02,40.69 68.58,43.13 IC2.8 71.19,43.18 v71.19,46.79 | v71.19,46.79
  Bottom 0.254: ENCODER_2.3 88.85,5.03 81.28,5.03 81.28,3.2 74.22,3.2 72.54,4.88 ENCODER_1.1 | v15.04,1.98 7.01,1.98 5.18,3.81 BLUETOOTH_1.1 | 71.19,47.97 71.19,62.16 IC1.8 71.83,68.02 71.83,70.87 | 71.19,47.97 | v71.19,46.79 71.19,47.97 | X102.40 62.79,76.2 65.05,73.94 65.05,70.87 71.83,70.87 | ULTRASOUND_1.1 72.39,20.22 71.02,21.59 v71.02,40.69 | 71.83,70.87 71.83,71.07 75.44,74.68 91.44,74.68 91.44,74.78 95.1,74.78 X103.40

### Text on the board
tPlace: AURIX™ Autonomous Robot 2018-2019 | Vcc | Vcc | GND | GND | Gaizi Amine / Bourgogne Marlon / Evaux Maxime / Nicolle Guillaume / Colrat Virgile | Vcc | Vcc | GND | Vcc | GND | GND | GND | Vcc | GND | Vcc | Vcc | GND | Vcc | GND | Vcc | GND | Vcc | Vcc | GND | GND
